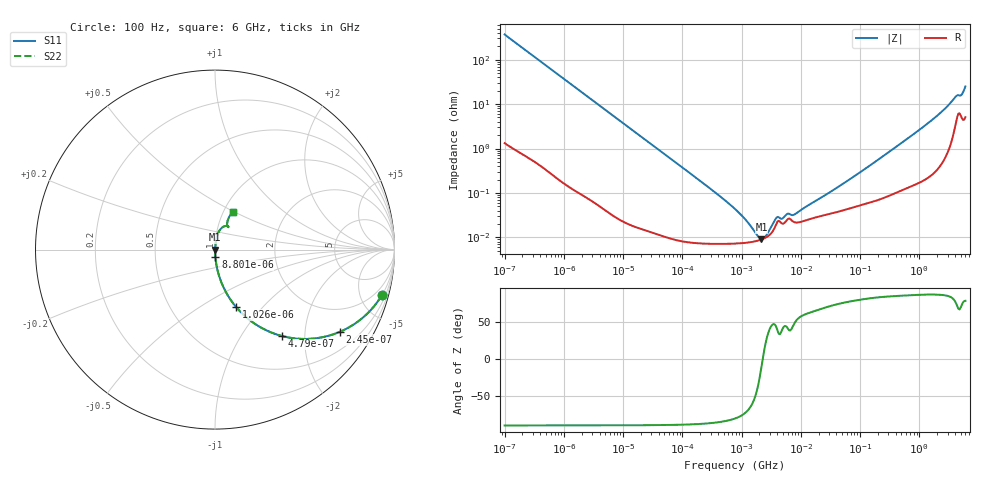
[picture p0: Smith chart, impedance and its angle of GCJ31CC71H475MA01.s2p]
!Murata Part Number: GCJ31CC71H475MA01
!These Parameters are Measured in Series Mode Connection
!Data Generated on Mar 13, 2026
!  o--ll--o
!Port1  Port2
!  o------o
!Operation Temp=25[degC], DC Bias Voltage=0[V]
!Freq. Start=100[Hz] Stop=6[GHz] 401[Steps]
# Hz S RI R 50
!Freq.(Hz) S11(Real) S11(Imag) S21(Real) S21(Imag) S12(Real) S12(Imag) S22(Real) S22(Imag)
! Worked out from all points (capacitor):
!   401 points, 100 Hz to 6 GHz, reference 50 ohm
!   read as one part in series: C = 4.31 uF near 109 Hz
!   lowest |Z| = 9.16 mohm at 2.169 MHz (marker M1)
!   series resonance near 2.28 MHz, so ESL is about 1.1 nH
!   S11 on the Smith chart (normalised r, x): 100 Hz: 1.03, -7.38; 245 Hz: 1.01, -3.02; 479 Hz: 1.01, -1.55; 1.026 kHz: 1.00, -0.72; 8.801 kHz: 1.00, -0.08; 6 GHz: 1.10, +0.49
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100  0.9308 -0.252  0.0692 0.252  0.0692 0.252  0.9308 -0.252
164  0.835 -0.3693  0.165 0.3693  0.165 0.3693  0.835 -0.3693
245  0.6944 -0.4586  0.3056 0.4586  0.3056 0.4586  0.6944 -0.4586
479  0.3746 -0.4818  0.6254 0.4818  0.6254 0.4818  0.3746 -0.4818
1026  0.1169 -0.3191  0.8831 0.3191  0.8831 0.3191  0.1169 -0.3191
2008  0.034 -0.1787  0.966 0.1787  0.966 0.1787  0.034 -0.1787
8801  0.00205 -0.0424  0.998 0.0424  0.998 0.0424  0.00205 -0.0424
40335  0.0002 -0.0093  0.9998 0.0093  0.9998 0.0093  0.0002 -0.0093
774597  7.28e-05 -0.000431  0.9999 0.000431  0.9999 0.000431  7.28e-05 -0.000431
1212075  7.61e-05 -0.000225  0.9999 0.000225  0.9999 0.000225  7.61e-05 -0.000225
1813585  8.36e-05 -7.77e-05  0.9999 7.77e-05  0.9999 7.77e-05  8.36e-05 -7.77e-05
2169299  9e-05 -1.7e-05  0.9999 1.7e-05  0.9999 1.7e-05  9e-05 -1.7e-05
2594782  0.0001 4.49e-05  0.9999 -4.49e-05  0.9999 -4.49e-05  0.0001 4.49e-05
3882480  0.000205 0.000187  0.9998 -0.000187  0.9998 -0.000187  0.000205 0.000187
6075234  0.000262 0.000223  0.9997 -0.000223  0.9997 -0.000223  0.000262 0.000223
7947587  0.000218 0.000251  0.9998 -0.000251  0.9998 -0.000251  0.000218 0.000251
1.555665e7  0.000269 0.000535  0.9997 -0.000535  0.9997 -0.000535  0.000269 0.000535
3.124326e8  0.000941 0.00844  0.9991 -0.00844  0.9991 -0.00844  0.000941 0.00844
1.791126e9  0.00516 0.0479  0.9948 -0.0479  0.9948 -0.0479  0.00516 0.0479
4.009986e9  0.0467 0.1278  0.9533 -0.1278  0.9533 -0.1278  0.0467 0.1278
5.016141e9  0.07 0.1286  0.93 -0.1286  0.93 -0.1286  0.07 0.1286
6e9  0.0975 0.2103  0.9025 -0.2103  0.9025 -0.2103  0.0975 0.2103
